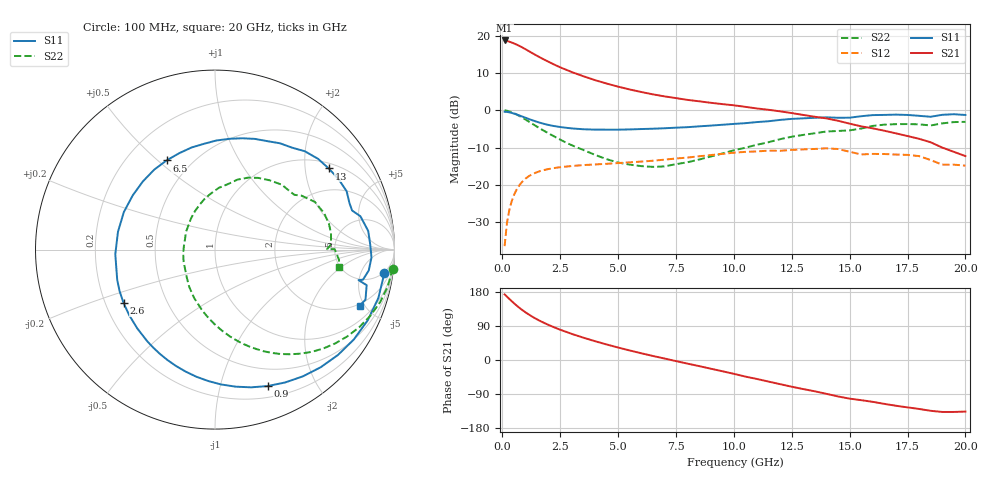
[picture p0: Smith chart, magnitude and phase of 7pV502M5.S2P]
! Infineon Technologies  Discrete & RF Semiconductors
! bfp620
! VCE = 0.50 V,  IC =  2.5 mA
! Common Emitter S-Parameters:  Sep 2002
# GHz  S  MA  R  50
!  f  S11  S21  S12  S22
! GHz  MAG  ANG  MAG  ANG  MAG  ANG  MAG  ANG
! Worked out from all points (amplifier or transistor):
!   59 points, 100 MHz to 20 GHz, reference 50 ohm
!   highest |S21| = 18.7 dB at 100 MHz (marker M1)
!   |S21| within 3 dB of that: start of sweep to 1.186 GHz
!   unconditionally stable (mu >= 1): 5.544 GHz to 11.8 GHz; 14.78 GHz to 15.53 GHz; 17.04 GHz to end of sweep
!   at 1 GHz: K = 0.21, MSG = 17.3 dB, |S12| = -18.3 dB
!   at 5.5 GHz: K = 1.00, MSG = 9.8 dB, |S12| = -14.0 dB
!   at 20 GHz: K = 1.95, MAG = -4.3 dB, |S12| = -14.9 dB
!   S11 on the Smith chart (normalised r, x): 100 MHz: 5, -13; 900 MHz: 0.31, -1.41; 2.6 GHz: 0.28, -0.25; 6.5 GHz: 0.37, +0.53; 13 GHz: 1.16, +2.67; 20 GHz: 1.87, -4.61
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0.1  0.9527 -7.9  8.6 173.2  0.0151 84.1  0.9955 -6.1
0.3  0.9378 -24.8  8.286 161.4  0.0456 75.3  0.9654 -17.6
0.5  0.9022 -40.6  7.856 150.0  0.0725 66.1  0.9126 -28.3
0.7  0.8592 -55.3  7.365 139.6  0.095 57.8  0.85 -37.9
0.9  0.815 -68.9  6.838 130.2  0.1133 50.5  0.7841 -46.6
1.1  0.7724 -81.4  6.308 121.8  0.1278 44.1  0.7189 -54.2
1.3  0.7334 -92.9  5.808 114.2  0.1391 38.6  0.6576 -61.1
1.7  0.6698 -113.3  4.963 101.0  0.155 29.8  0.5528 -72.8
2.2  0.6165 -134.7  4.15 87.3  0.1674 21.6  0.4528 -85.1
2.6  0.5902 -149.6  3.644 77.7  0.1739 16.4  0.3891 -94.4
3  0.5704 -162.8  3.244 68.9  0.1789 11.9  0.3397 -103.0
3.5  0.556 -177.4  2.854 58.9  0.1842 7.3  0.2933 -113.4
5  0.549 146.6  2.07 32.9  0.1959 -2.7  0.1992 -146.7
6.5  0.5654 118.5  1.632 10.7  0.2105 -10.8  0.1743 173.4
7  0.573 110.3  1.534 4.0  0.2176 -13.3  0.1768 161.1
8.5  0.6079 89.3  1.317 -16.1  0.2417 -22.2  0.2183 128.0
10.5  0.6707 64.3  1.109 -43.8  0.2768 -38.7  0.3148 93.8
13  0.7784 35.5  0.864 -76.8  0.2989 -60.9  0.467 58.8
13.5  0.7924 29.8  0.817 -82.6  0.3027 -65.8  0.4919 51.7
15  0.7944 15.9  0.661 -101.9  0.2776 -86.2  0.5372 34.6
17  0.873 -2.9  0.49 -120.7  0.2549 -97.0  0.6508 12.9
20  0.8639 -21.2  0.243 -136.1  0.1809 -115.3  0.6987 -8.2
